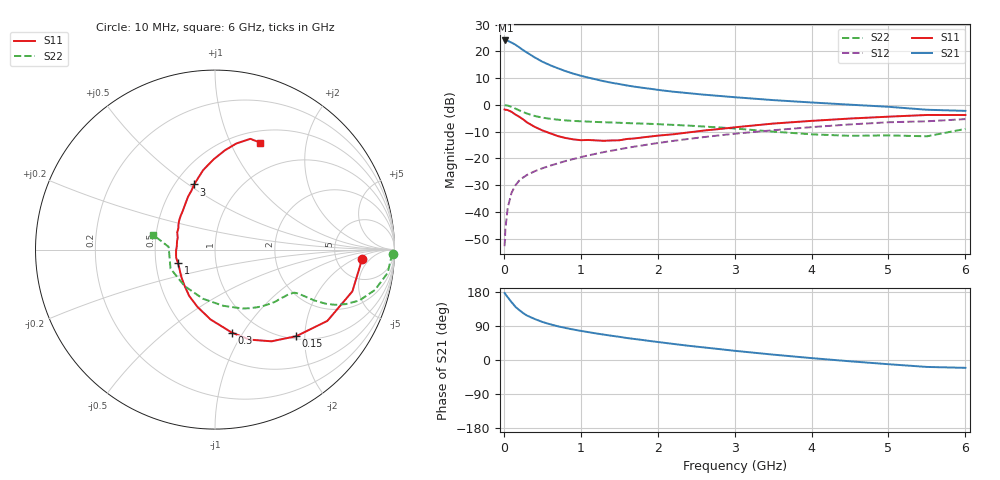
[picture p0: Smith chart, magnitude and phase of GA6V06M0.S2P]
! Infineon Technologies  Discrete & RF Semiconductors
! BF775
! Si NPN RF Bipolar Junction Transistor in SOT23
! VCE = 6 V  IC = 6 mA
! Common Emitter S-Parameters:  May  1996
# GHz  S  MA  R  50
!  f  S11  S21  S12  S22
! GHz  MAG  ANG  MAG  ANG  MAG  ANG  MAG  ANG
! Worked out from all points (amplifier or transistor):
!   36 points, 10 MHz to 6 GHz, reference 50 ohm
!   highest |S21| = 24.1 dB at 20 MHz (marker M1)
!   |S21| within 3 dB of that: start of sweep to 221.5 MHz
!   unconditionally stable (mu >= 1): 773.2 MHz to 3.065 GHz
!   at 250 MHz: K = 0.52, MSG = 23.8 dB, |S12| = -27.1 dB
!   at 1.4 GHz: K = 1.11, MAG = 10.7 dB, |S12| = -17.1 dB
!   at 6 GHz: K = 0.92, MSG = 1.5 dB, |S12| = -5.3 dB
!   S11 on the Smith chart (normalised r, x): 10 MHz: 9.26, -2.84; 150 MHz: 1.06, -1.81; 300 MHz: 0.75, -0.89; 1 GHz: 0.65, -0.10; 3 GHz: 0.62, +0.53; 6 GHz: 0.64, +1.30
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0.01  0.8204 -3.5  15.9 176.8  0.0023 90.2  0.9921 -1.4
0.02  0.8122 -6.9  15.96 173.8  0.0048 85.3  0.9815 -3.1
0.05  0.8 -16.9  15.7 165.6  0.0119 81.4  0.9705 -7.7
0.1  0.7414 -32.4  14.56 152.8  0.0228 74.0  0.9186 -14.2
0.15  0.6616 -46.8  13.3 140.5  0.0314 67.6  0.8529 -19.4
0.2  0.6 -58.4  11.88 131.8  0.0386 64.0  0.7901 -22.6
0.25  0.5371 -69.0  10.57 123.9  0.044 61.2  0.7359 -24.7
0.3  0.472 -78.5  9.488 117.4  0.0491 60.4  0.6894 -26.0
0.4  0.3898 -93.7  7.723 108.3  0.0575 59.1  0.6216 -27.1
0.5  0.3339 -107.0  6.405 100.5  0.0654 59.1  0.5783 -27.4
0.6  0.2956 -119.1  5.522 94.4  0.0732 59.2  0.551 -27.6
0.8  0.2411 -141.2  4.28 84.6  0.0893 60.3  0.5137 -28.1
1  0.2192 -160.5  3.503 76.9  0.1056 60.8  0.4943 -29.4
1.1  0.2212 -168.4  3.223 73.5  0.1141 60.8  0.487 -30.5
1.3  0.2135 175.6  2.766 67.0  0.1313 60.7  0.474 -32.4
1.6  0.231 155.6  2.304 58.0  0.1573 59.7  0.4568 -36.3
2.2  0.2823 129.2  1.764 42.5  0.2124 56.0  0.4233 -46.4
3  0.381 107.8  1.391 24.3  0.2892 48.7  0.3621 -65.0
3.5  0.4477 98.5  1.228 14.2  0.3361 43.0  0.3167 -81.5
4.5  0.5559 84.3  1.009 -3.4  0.4316 30.6  0.2645 -129.8
5.5  0.6479 72.3  0.811 -18.3  0.4938 15.5  0.2588 176.6
6  0.6468 67.0  0.773 -20.7  0.5427 11.4  0.3558 166.5
